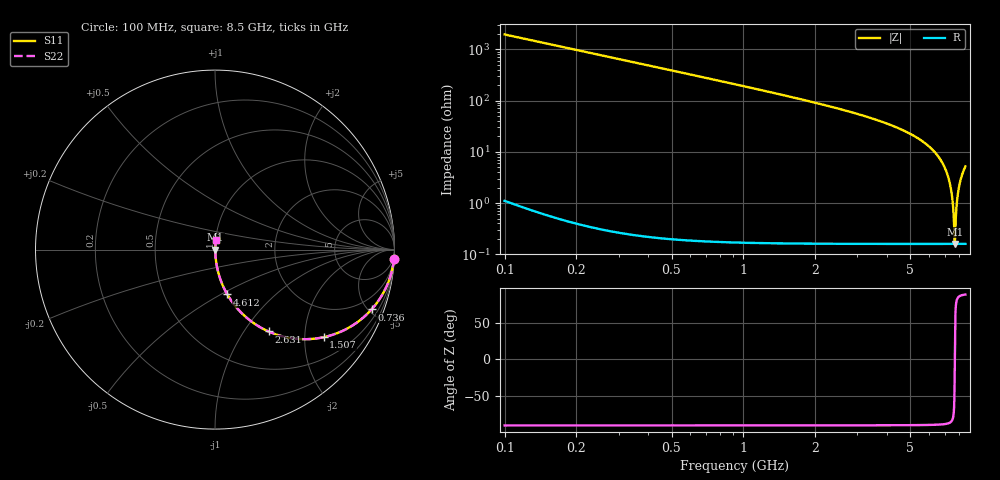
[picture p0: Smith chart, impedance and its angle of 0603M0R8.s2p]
! Created Wed Apr 18 12:01:52 2012
# hz S ma R 50
! 2 Port Network Data from SP1.SP block
! freq  magS11  angS11  magS21  angS21  magS12  angS12  magS22  angS22
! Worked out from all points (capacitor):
!   8401 points, 100 MHz to 8.5 GHz, reference 50 ohm
!   read as one part in series: C = 820 fF near 142 MHz
!   lowest |Z| = 160 mohm at 7.674 GHz (marker M1)
!   series resonance near 7.674 GHz, so ESL is about 520 pH
!   S11 on the Smith chart (normalised r, x): 100 MHz: 1, -39; 736 MHz: 1.00, -5.23; 1.507 GHz: 1.00, -2.48; 2.631 GHz: 1.00, -1.30; 4.612 GHz: 1.00, -0.54; 8.5 GHz: 1.00, +0.10
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1e8  0.9986 -2.9  0.05146 87.0  0.05146 87.0  0.9986 -2.9
3.38e8  0.985 -9.9  0.1719 80.1  0.1719 80.1  0.985 -9.9
7.36e8  0.9337 -20.9  0.3574 69.0  0.3574 69.0  0.9337 -20.9
1.5e9  0.779 -38.8  0.626 51.2  0.626 51.2  0.779 -38.8
1.507e9  0.7775 -38.9  0.6279 51.0  0.6279 51.0  0.7775 -38.9
2.631e9  0.545 -56.8  0.8371 33.0  0.8371 33.0  0.545 -56.8
2.9e9  0.4971 -60.0  0.8663 29.8  0.8663 29.8  0.4971 -60.0
4.3e9  0.2955 -72.5  0.9538 17.2  0.9538 17.2  0.2955 -72.5
4.612e9  0.2594 -74.6  0.9642 15.0  0.9642 15.0  0.2594 -74.6
5.7e9  0.1508 -80.7  0.987 8.7  0.987 8.7  0.1508 -80.7
6.543e9  0.08071 -84.2  0.9951 4.6  0.9951 4.6  0.08071 -84.2
7.1e9  0.03936 -85.4  0.9976 2.3  0.9976 2.3  0.03936 -85.4
7.319e9  0.02402 -84.8  0.9981 1.4  0.9981 1.4  0.02402 -84.8
7.474e9  0.01346 -82.4  0.9983 0.8  0.9983 0.8  0.01346 -82.4
7.564e9  0.007488 -77.3  0.9984 0.4  0.9984 0.4  0.007488 -77.3
7.647e9  0.002404 -48.3  0.9984 0.1  0.9984 0.1  0.002404 -48.3
7.674e9  0.001597 -0.5  0.9984 0.0  0.9984 0.0  0.001597 -0.5
7.7e9  0.002329 46.6  0.9984 -0.1  0.9984 -0.1  0.002329 46.6
7.799e9  0.008312 78.5  0.9984 -0.5  0.9984 -0.5  0.008312 78.5
7.931e9  0.01672 83.6  0.9983 -1.0  0.9983 -1.0  0.01672 83.6
8.166e9  0.03146 85.3  0.9979 -1.8  0.9979 -1.8  0.03146 85.3
8.5e9  0.05174 85.3  0.9971 -3.0  0.9971 -3.0  0.05174 85.3
